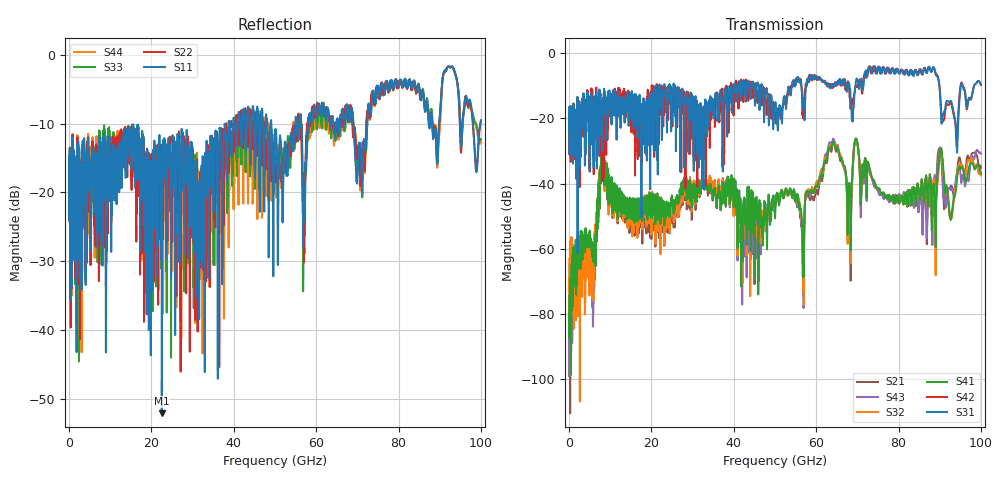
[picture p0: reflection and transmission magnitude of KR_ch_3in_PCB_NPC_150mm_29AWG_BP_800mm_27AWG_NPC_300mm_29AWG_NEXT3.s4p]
# GHz S RI R 45
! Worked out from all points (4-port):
!   4000 points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, 25 MHz to 100 GHz, reference 45 ohm
!   strongest paths, dB at 25 MHz, 25.02 GHz, 50.02 GHz, 75.03 GHz, 100 GHz:
!     S31: -21.3, -14.8, -15.8, -5.1, -9.6
!     S42: -21.3, -17.5, -18.0, -4.3, -9.8
!     S41: -87.0, -45.6, -50.5, -41.7, -37.0
!     S32: -86.5, -47.2, -47.4, -41.7, -37.5
!     S43: -88.6, -47.5, -46.3, -42.2, -30.8
!     S21: -94.7, -50.3, -47.2, -42.1, -35.1
!   lowest |S11| = -52.1 dB at 22.52 GHz (marker M1), VSWR 1.00, Z = 45 + j0.221 ohm
!   |S11| at or under -10 dB: start of sweep to 38.73 GHz; 49.12 GHz to 54.96 GHz (5.844 GHz wide, 11.2 % of centre); 69.04 GHz to 72.39 GHz (3.354 GHz wide, 4.74 % of centre)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
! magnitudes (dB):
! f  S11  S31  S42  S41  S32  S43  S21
! 25 MHz  -16.7  -21.3  -21.3  -87.0  -86.5  -88.6  -94.7
! 5.875 GHz  -16.9  -19.7  -14.4  -61.9  -69.7  -80.1  -76.9
! 8.25 GHz  -12.8  -14.6  -18.7  -32.4  -32.6  -32.3  -32.9
! 22.52 GHz  -52.1  -23.4  -11.1  -48.2  -53.0  -48.8  -52.1
! 56.67 GHz  -16.7  -14.9  -18.9  -58.9  -58.9  -60.0  -58.1
! 63.85 GHz  -9.2  -9.6  -10.1  -28.4  -28.4  -27.4  -29.3
! 100 GHz  -9.5  -9.6  -9.8  -37.0  -37.5  -30.8  -35.1
